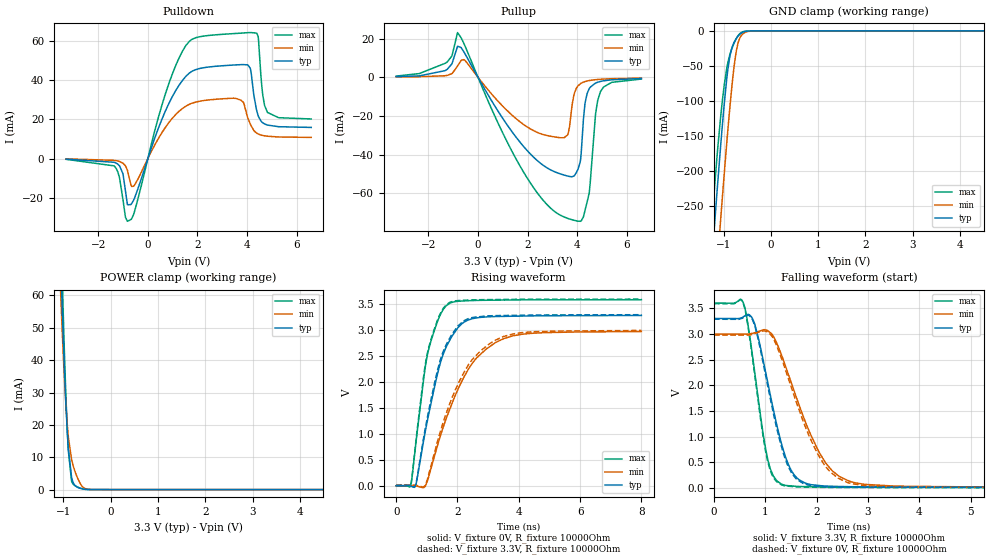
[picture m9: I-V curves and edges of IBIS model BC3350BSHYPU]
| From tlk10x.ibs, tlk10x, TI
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|   Model
[Model]   BC3350BSHYPU
Model_type   I/O
Polarity   Non-Inverting
Enable   Active-Low
Vinl = 0.99
Vinh = 2.31
Vmeas = 1.65
Vref = 1.65
Cref = 1pF
Rref = 10000
|   typ   min   max
C_comp   1.913pF   1.872pF   1.989pF
[Voltage Range]   3.3   3   3.6
[Temperature Range]   25   125   -40
[Pullup Reference]   3.3   3   3.6
[Pulldown Reference]   -0   -0   -0
[Power Clamp Reference]   3.3   3   3.6
[GND Clamp Reference]   -0   -0   -0
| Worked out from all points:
|   slope of the pulldown table from 0 to 0.495 V, typ, clamps not added: 27.8 ohm
|   slope of the pullup table from 0 to 0.495 V, typ, clamps not added: 45 ohm
|   GND clamp passes 1 mA (typ) near -0.55 V on its own axis
|   POWER clamp passes 1 mA (typ) near -0.73 V on its own axis
|   falling waveform, V_fixture 3.3V, R_fixture 10000Ohm: 20-80 % time 447ps typ, 717ps min, 307ps max; typ from 3.3 V to 0.011 V
|   rising waveform, V_fixture 0V, R_fixture 10000Ohm: 20-80 % time 762ps typ, 1.25ns min, 554ps max; typ from 0.003 V to 3.29 V
|   rising waveform, V_fixture 3.3V, R_fixture 10000Ohm: 20-80 % time 748ps typ, 1.2ns min, 550ps max; typ from 0.011 V to 3.3 V
|   falling waveform, V_fixture 0V, R_fixture 10000Ohm: 20-80 % time 439ps typ, 696ps min, 302ps max; typ from 3.29 V to 0.003 V
[Pulldown]
|   Voltage   I(typ)   I(min)   I(max)
-3.3V     -306.9uA   -177.2uA   -405.9uA
-1.36V    -1.92mA    -935.2uA   -3.758mA
-904.2mV  -16.6mA    -3.769mA   -30.08mA
-686.4mV  -23.56mA   -13.42mA   -31.2mA
976.8mV   31.41mA    20.44mA    42.88mA
2.224V    46.37mA    29.58mA    62.55mA
3.749V    47.99mA    29.83mA    64.09mA
4.036V    47.8mA     20.63mA    64.34mA
4.392V    24.4mA     12.94mA    64.04mA
4.64V     18.21mA    11.76mA    31.97mA
4.818V    17.14mA    11.41mA    23.72mA
6.59V     15.9mA     10.79mA    20.22mA
[GND Clamp]
|   Voltage   I(typ)   I(min)   I(max)
-3.3V     -2.327A    -2.431A    -2.267A
-1.251V   -331.9mA   -441.7mA   -275.1mA
-1.142V   -233.8mA   -342.1mA   -183.1mA
-1.063V   -165.8mA   -271.4mA   -124.1mA
-993.3mV  -110.6mA   -211.3mA   -81.89mA
-933.9mV  -69.67mA   -161.9mA   -54.4mA
-864.6mV  -35.74mA   -108.2mA   -33.51mA
-795.3mV  -19.21mA   -61.63mA   -20.46mA
-735.9mV  -11.6mA    -31.59mA   -11.84mA
-676.5mV  -6.34mA    -13.94mA   -5.581mA
-597.3mV  -2.203mA   -4.7mA     -1.435mA
6.59V     0A         0A         0A
[Pullup]
|   Voltage   I(typ)   I(min)   I(max)
-3.3V     399.3uA    220.7uA    636uA
-1.251V   4.083mA    981.6uA    7.893mA
-825mV    16.09mA    5.869mA    23.18mA
1.531V    -30.93mA   -21.37mA   -42.19mA
3.214V    -49.54mA   -31.12mA   -70.62mA
3.62V     -51.15mA   -29.63mA   -73.07mA
3.868V    -51.13mA   -9.195mA   -74.03mA
4.125V    -43.73mA   -3.369mA   -74.58mA
4.402V    -8.37mA    -1.906mA   -64.53mA
4.749V    -2.951mA   -1.219mA   -18.4mA
4.937V    -2.145mA   -1.017mA   -7.525mA
6.59V     -611.9uA   -409.7uA   -889.9uA
[POWER Clamp]
|   Voltage   I(typ)   I(min)   I(max)
-3.3V     1.546A     1.464A     1.615A
-1.053V   70.22mA    59.7mA     81.97mA
-1.023V   56.54mA    49.09mA    65.65mA
-1.013V   52.23mA    45.76mA    60.44mA
-943.8mV  26.11mA    25.95mA    28.51mA
-894.3mV  12.79mA    16.42mA    12.2mA
-825mV    3.776mA    9.362mA    2.627mA
-775.5mV  1.732mA    6.644mA    1.49mA
-686.4mV  636.8uA    3.184mA    717.6uA
-567.6mV  166.1uA    574.9uA    153.8uA
-409.2mV  18.69uA    30.27uA    21.29uA
6.59V     0A         0A         0A
[Ramp]
R_load = 10000
|   typ   min   max
dV/dt_r   1.96965/7.63167e-10   1.78363/1.24727e-09   2.15149/5.53498e-10
dV/dt_f   1.97323/4.46974e-10   1.78829/7.13277e-10   2.15441/3.05658e-10
[Falling Waveform]
V_fixture = 3.3V
V_fixture_min = 3V
V_fixture_max = 3.6V
R_fixture = 10000Ohm
C_fixture = 0F
|   Time   V(typ)   V(min)   V(max)
0s        3.3V       2.996V     3.6V
573.2ps   3.334V     2.995V     3.598V
791.9ps   3.194V     3.022V     2.259V
1.036ns   2.103V     3.068V     603.2mV
1.15ns    1.554V     2.961V     243.1mV
1.315ns   862.7mV    2.59V      75.23mV
1.608ns   203.5mV    1.755V     31.65mV
2.043ns   48.69mV    707.8mV    21.21mV
2.629ns   25.66mV    135.4mV    16.77mV
8ns       10.9mV     15.42mV    9.3mV
[Rising Waveform]
V_fixture = 0V
V_fixture_min = 0V
V_fixture_max = 0V
R_fixture = 10000Ohm
C_fixture = 0F
|   Time   V(typ)   V(min)   V(max)
0s        2.598mV    3.737mV    2.622mV
461ps     -2.513mV   4.706mV    -12.24mV
632.9ps   5.736mV    2.935mV    771.3mV
1.029ns   1.289V     114.9mV    2.554V
1.392ns   2.264V     868.9mV    3.236V
1.633ns   2.678V     1.301V     3.473V
2.008ns   3.045V     1.852V     3.558V
2.464ns   3.22V      2.348V     3.572V
3.495ns   3.267V     2.836V     3.582V
8ns       3.285V     2.976V     3.588V
[Rising Waveform]
V_fixture = 3.3V
V_fixture_min = 3V
V_fixture_max = 3.6V
R_fixture = 10000Ohm
C_fixture = 0F
|   Time   V(typ)   V(min)   V(max)
0s        10.9mV     15.41mV    9.3mV
461ps     5.575mV    16.24mV    -3.793mV
623.1ps   4.801mV    16.03mV    754.6mV
1.02ns    1.328V     132.5mV    2.566V
1.354ns   2.243V     871.9mV    3.206V
1.633ns   2.722V     1.398V     3.491V
2.008ns   3.078V     1.952V     3.572V
2.464ns   3.242V     2.422V     3.584V
3.495ns   3.284V     2.878V     3.594V
8ns       3.3V       2.996V     3.6V
[Falling Waveform]
|Gnd
V_fixture = 0V
V_fixture_min = 0V
V_fixture_max = 0V
R_fixture = 10000Ohm
C_fixture = 0F
|   Time   V(typ)   V(min)   V(max)
0s        3.285V     2.976V     3.588V
573.2ps   3.32V      2.976V     3.581V
791.9ps   3.165V     3.006V     2.207V
1.029ns   2.077V     3.043V     594.6mV
1.144ns   1.512V     2.928V     227.6mV
1.315ns   804.7mV    2.523V     60.97mV
1.608ns   172mV      1.66V      22.81mV
2ns       34.26mV    702.2mV    13.57mV
2.578ns   16.65mV    115.8mV    8.725mV
8ns       2.599mV    3.742mV    2.623mV
